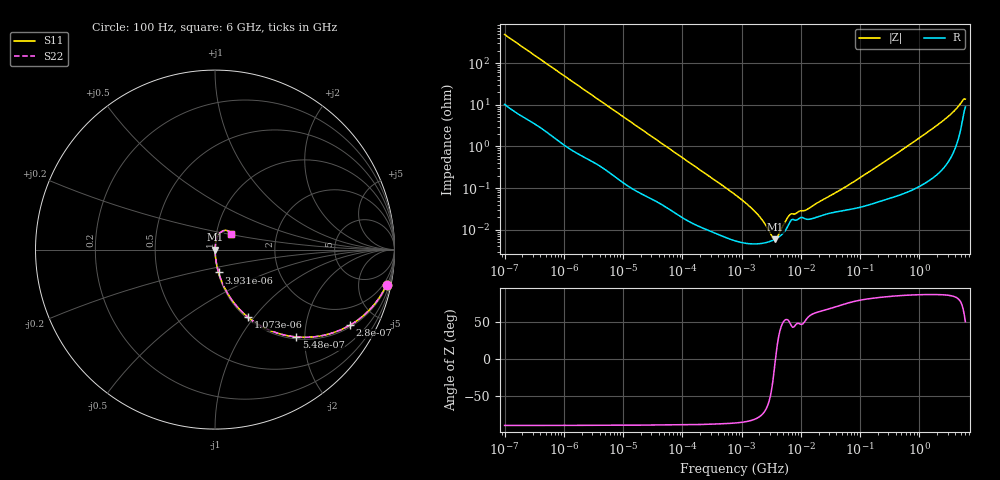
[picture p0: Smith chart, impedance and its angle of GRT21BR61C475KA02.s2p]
!Murata Part Number: GRT21BR61C475KA02
!These Parameters are Measured in Series Mode Connection
!Data Generated on Jun 19, 2026
!  o--ll--o
!Port1  Port2
!  o------o
!Operation Temp=25[degC], DC Bias Voltage=0[V]
!Freq. Start=100[Hz] Stop=6[GHz] 401[Steps]
# Hz S RI R 50
!Freq.(Hz) S11(Real) S11(Imag) S21(Real) S21(Imag) S12(Real) S12(Imag) S22(Real) S22(Imag)
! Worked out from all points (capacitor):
!   401 points, 100 Hz to 6 GHz, reference 50 ohm
!   read as one part in series: C = 3.26 uF near 109 Hz
!   lowest |Z| = 5.96 mohm at 3.712 MHz (marker M1)
!   series resonance near 3.738 MHz, so ESL is about 560 pH
!   S11 on the Smith chart (normalised r, x): 100 Hz: 1.20, -9.73; 280 Hz: 1.08, -3.52; 548 Hz: 1.04, -1.82; 1.073 kHz: 1.02, -0.94; 3.931 kHz: 1.01, -0.26; 6 GHz: 1.18, +0.21
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100  0.9557 -0.1955  0.0443 0.1955  0.0443 0.1955  0.9557 -0.1955
164  0.8944 -0.2972  0.1056 0.2972  0.1056 0.2972  0.8944 -0.2972
280  0.7508 -0.4216  0.2492 0.4216  0.2492 0.4216  0.7508 -0.4216
548  0.4529 -0.4866  0.5471 0.4866  0.5471 0.4866  0.4529 -0.4866
1073  0.1848 -0.3775  0.8152 0.3775  0.8152 0.3775  0.1848 -0.3775
2008  0.0645 -0.2341  0.9355 0.2341  0.9355 0.2341  0.0645 -0.2341
3931  0.0199 -0.1271  0.9801 0.1271  0.9801 0.1271  0.0199 -0.1271
40335  0.000613 -0.0132  0.9994 0.0132  0.9994 0.0132  0.000613 -0.0132
774597  5.48e-05 -0.000699  0.9999 0.000699  0.9999 0.000699  5.48e-05 -0.000699
1658239  4.58e-05 -0.000276  1 0.000276  1 0.000276  4.58e-05 -0.000276
2837864  5.1e-05 -8.57e-05  0.9999 8.57e-05  0.9999 8.57e-05  5.1e-05 -8.57e-05
3712478  5.96e-05 -2.1e-06  0.9999 2.1e-06  0.9999 2.1e-06  5.96e-05 -2.1e-06
4643984  7.4e-05 6.9e-05  0.9999 -6.9e-05  0.9999 -6.9e-05  7.4e-05 6.9e-05
6644369  0.000158 0.000173  0.9998 -0.000173  0.9998 -0.000173  0.000158 0.000173
1.189169e7  0.000183 0.000228  0.9998 -0.000228  0.9998 -0.000228  0.000183 0.000228
1.555665e7  0.000185 0.00032  0.9998 -0.00032  0.9998 -0.00032  0.000185 0.00032
6.233367e7  0.000302 0.00112  0.9997 -0.00112  0.9997 -0.00112  0.000302 0.00112
3.124326e8  0.00059 0.00512  0.9994 -0.00512  0.9994 -0.00512  0.00059 0.00512
2.240541e9  0.00376 0.0362  0.9962 -0.0362  0.9962 -0.0362  0.00376 0.0362
4.385646e9  0.0193 0.0819  0.9807 -0.0819  0.9807 -0.0819  0.0193 0.0819
5.245841e9  0.0462 0.1052  0.9538 -0.1052  0.9538 -0.1052  0.0462 0.1052
6e9  0.0896 0.0877  0.9104 -0.0877  0.9104 -0.0877  0.0896 0.0877
